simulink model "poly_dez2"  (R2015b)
settings: Solver=VariableStepAuto  StartTime=0.0  StopTime=15  RelTol=1e-3
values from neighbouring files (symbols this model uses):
  g = firpolyphase(hdez, M)    [poly_dez_1.m]    (also in poly_dez_2.m; poly_interp_1.m = firpolyphase(hint, L); poly_interp_2.m = firpolyphase(hint, L))
  hdez = fir1(nord2, 1/M)    [poly_dez_1.m]    (also in poly_dez_2.m)
  hTP = fir1(nord, 2*fp/fs)    [dezimier_2.m]    (also in dezimier_3.m; frac_delay_1.m = fir1(nord, fp*2); frac_delay_2.m = fir1(nord, fp*2); lagrange_3.m = fir1(40, 0.5))
  M = 5    [dezimier_1.m]    (also in dezimier_11.m; dezimier_2.m; dezimier_3.m; farrow_3.m)
  Ts = 1/fs    (= 5e-05)    [basisband_1.m]    (also in basisband_2.m = 5e-06; dezimier_1.m = 0.0005; dezimier_11.m = 0.0005; dezimier_2.m = 0.0005)
libraries: simulink x1

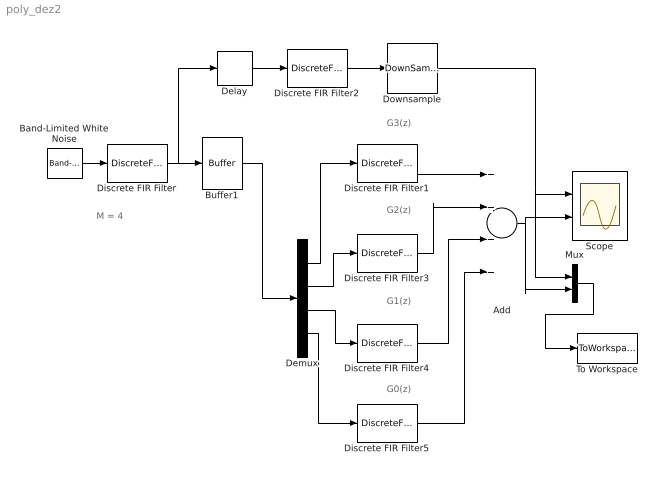
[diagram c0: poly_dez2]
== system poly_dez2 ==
  note: G0(z)
  note: G1(z)
  note: G2(z)
  note: G3(z)
  note: M = 4
  Add : Sum  Inputs=++++
  Band-Limited White Noise : simulink/Sources/Band-Limited White Noise  Cov=Ts  Ts=Ts  seed=[23341]
  Buffer1 : Buffer  N=M  TreatMby1Signals=One channel  OutputFrames=off
  Delay : Delay  DelayLength=1
  Demux : Demux
  Discrete FIR Filter : DiscreteFir  Coefficients=hTP
  Discrete FIR Filter1 : DiscreteFir  Coefficients=(g(4,:))
  Discrete FIR Filter2 : DiscreteFir  Coefficients=hdez
  Discrete FIR Filter3 : DiscreteFir  Coefficients=(g(3,:))
  Discrete FIR Filter4 : DiscreteFir  Coefficients=(g(2,:))
  Discrete FIR Filter5 : DiscreteFir  Coefficients=(g(1,:))
  Downsample : DownSample  N=4  RateOptions=Allow multirate processing
  Mux : Mux  Inputs=2
  Scope : Scope  NumInputPorts=2
  To Workspace : ToWorkspace  VariableName=y  SaveFormat=Timeseries  SampleTime=-1
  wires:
  Band-Limited White Noise/1 -> Discrete FIR Filter/1
  Discrete FIR Filter1/1 -> Add/1
  Discrete FIR Filter3/1 -> Add/2
  Discrete FIR Filter4/1 -> Add/3
  Add/1 -> Mux/2, Scope/2
  Discrete FIR Filter5/1 -> Add/4
  Downsample/1 -> Mux/1, Scope/1
  Discrete FIR Filter/1 -> Delay/1, Buffer1/1
  Demux/4 -> Discrete FIR Filter5/1
  Demux/1 -> Discrete FIR Filter1/1
  Demux/3 -> Discrete FIR Filter4/1
  Demux/2 -> Discrete FIR Filter3/1
  Buffer1/1 -> Demux/1
  Discrete FIR Filter2/1 -> Downsample/1
  Delay/1 -> Discrete FIR Filter2/1
  Mux/1 -> To Workspace/1
